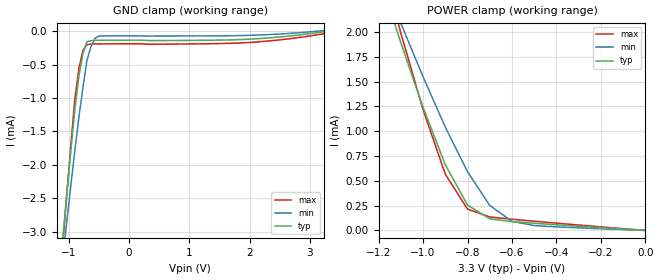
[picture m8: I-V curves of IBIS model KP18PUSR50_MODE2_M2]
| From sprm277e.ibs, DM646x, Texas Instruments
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|   Model Cell KP18PUSR50_MODE2_M2
[Model]   KP18PUSR50_MODE2_M2
Model_type   Input
Polarity   Non-Inverting
Vinl =  0.8V
Vinh =  2V
C_comp   0.7641276p   0.7025916p   0.8394225p
[Model Spec]
Vinl   0.8V   0.8V   0.8V
Vinh   2V   2V   2V
[Temperature Range]   25   105   0
[Voltage Range]   3.3   3.14   3.47
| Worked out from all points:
|   GND clamp passes 1 mA (typ) near -0.88 V on its own axis
|   POWER clamp passes 1 mA (typ) near -0.96 V on its own axis
[POWER_clamp]
|   voltage   I(typ)   I(min)   I(max)
-3.3V     17.71mA    14.67mA    20.82mA
-1.133V   2.126mA    2.273mA    2.272mA
-1.1V     1.894mA    2.088mA    1.99mA
-1.067V   1.676mA    1.909mA    1.733mA
-1V       1.241mA    1.55mA     1.218mA
-900mV    663.2uA    1.042mA    567.9uA
-800mV    255.8uA    591.9uA    215uA
-700mV    117.5uA    252.4uA    136.6uA
-600mV    89.09uA    91.71uA    113.3uA
-500mV    72.99uA    49.44uA    93.38uA
0V        95.23nA    66.33nA    458.2nA
[GND_clamp]
|   voltage   I(typ)   I(min)   I(max)
-3.3V     -26.2mA    -22.27mA   -29.13mA
-1.1V     -3.083mA   -3.375mA   -3.167mA
-1.033V   -2.417mA   -2.83mA    -2.409mA
-900mV    -1.156mA   -1.771mA   -1.002mA
-833.3mV  -666.4uA   -1.283mA   -553.5uA
-766.7mV  -333.7uA   -838uA     -287uA
-700mV    -157.8uA   -435.3uA   -203uA
-633.3mV  -144.6uA   -227.6uA   -195.7uA
-566.7mV  -137.7uA   -107.3uA   -191.9uA
-500mV    -137.1uA   -74.15uA   -191.4uA
1.833V    -127.3uA   -67.09uA   -177.5uA
3.233V    -8.718uA   8.017uA    -38.34uA
